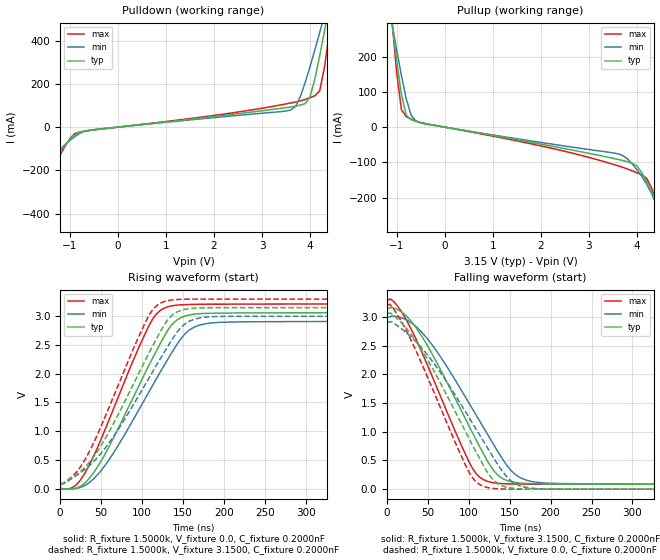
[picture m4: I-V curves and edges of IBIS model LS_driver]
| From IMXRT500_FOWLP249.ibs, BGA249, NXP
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[Model] LS_driver
|   Model LS_driver
| Library cells for typ/min/max conditions are connected as defined below:
|  pad_usbdp - External Pad
|  usb2_tx_d_data_dp - Core Input
|  gnda - gnda
|  pad_usb_vss - pad_usb_vss
|  usb2_reg_tx_fs_hiz - gnda
|  usb2_reg_tx_hs_term - gnda
|  usb2_reg_tx_hs_xcvr - gnda
|  usb2_reg_tx_ls_en - vddd
|  usbphy_d2a_txhsactive - gnda
|  vddb - vddb
|  vddd - vddd
| All other pins connected to ground
Model_type Output
Polarity   Non-Inverting
Enable   Active-Low
C_comp   2.8431pF   2.6338pF   3.0727pF
[Temperature Range]   27.0000   0.1250k   -40.0000
[Voltage Range]   3.1500V   3.0000V   3.3000V
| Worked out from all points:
|   slope of the pulldown table from 0 to 0.472 V, typ, clamps not added: 41.5 ohm
|   slope of the pullup table from 0 to 0.472 V, typ, clamps not added: 42.2 ohm
|   rising waveform, R_fixture 1.5000k, V_fixture 0.0, C_fixture 0.2000nF: 20-80 % time 64.1ns typ, 71.2ns min, 56.3ns max; typ from 0 V to 3.06 V
|   rising waveform, R_fixture 1.5000k, V_fixture 3.1500, C_fixture 0.2000nF: 20-80 % time 67.1ns typ, 75.8ns min, 57.7ns max; typ from 0.085 V to 3.15 V
|   falling waveform, R_fixture 1.5000k, V_fixture 3.1500, C_fixture 0.2000nF: 20-80 % time 66.8ns typ, 74.8ns min, 58ns max; typ from 3.15 V to 0.085 V
|   falling waveform, R_fixture 1.5000k, V_fixture 0.0, C_fixture 0.2000nF: 20-80 % time 68.9ns typ, 78.6ns min, 58.5ns max; typ from 3.06 V to 0 V
[Pulldown]
|Voltage   I(typ)   I(min)   I(max)
-3.3V     -1.789A    -1.328A    -2.415A
-2V       -541mA     -458.4mA   -672.7mA
-1.8V     -385mA     -344.5mA   -475.2mA
-1.2V     -110.9mA   -103.2mA   -128.7mA
-700mV    -18.35mA   -19.33mA   -19.54mA
3.6V      93.13mA    79.46mA    111.7mA
4V        140.3mA    280mA      135.9mA
4.2V      328.8mA    437.3mA    167.5mA
4.3V      443.1mA    519.1mA    276.2mA
4.4V      562.1mA    602.3mA    433.8mA
4.5V      683.9mA    686.7mA    605.7mA
6.6V      3.469A     2.552A     4.733A
[Pullup]
|Voltage   I(typ)   I(min)   I(max)
-3.3V     3.149A     2.232A     4.536A
-1.1V     298.4mA    297.3mA    309.5mA
-1V       188.4mA    219.5mA    155mA
-900mV    91.83mA    145.9mA    49.27mA
-800mV    33.62mA    80.51mA    29.57mA
-700mV    21.24mA    34.27mA    23.01mA
-400mV    9.525mA    9.075mA    10.13mA
3.7V      -94.61mA   -80.02mA   -113.9mA
4V        -110.4mA   -120.8mA   -129.3mA
4.2V      -153.7mA   -161.4mA   -144.6mA
4.6V      -279.6mA   -298.9mA   -297.9mA
6.6V      -2.055A    -1.587A    -2.608A
[Ramp]
| variable   typ   min   max
dV/dt_r  0.9799/85.9935n   0.8933/97.2090n   1.0678/74.5644n
dV/dt_f  0.9878/89.0736n   0.8995/0.1028u   1.0749/76.7496n
R_load = 45.0000
[Rising Waveform]
R_fixture= 1.5000k
V_fixture= 0.0
V_fixture_min= 0.0
V_fixture_max= 0.0
C_fixture= 0.2000nF
|time   V(typ)   V(min)   V(max)
0s        172.1nV    5.49uV     121.3nV
19.94ns   10.73mV    2.415mV    71.03mV
40.93ns   278.8mV    171.3mV    568mV
66.15ns   913.6mV    644.9mV    1.428V
107ns     2.113V     1.653V     2.8V
117.3ns   2.398V     1.912V     3.039V
135.3ns   2.837V     2.348V     3.179V
157.1ns   3.022V     2.758V     3.206V
193.4ns   3.055V     2.893V     3.211V
1us       3.064V     2.913V     3.215V
[Rising Waveform]
R_fixture= 1.5000k
V_fixture= 3.1500
V_fixture_min= 3.0000
V_fixture_max= 3.3000
C_fixture= 0.2000nF
|time   V(typ)   V(min)   V(max)
0s        84.94mV    86.28mV    83.78mV
22.75ns   274.8mV    254.3mV    338.8mV
47.41ns   691.8mV    573.5mV    1.002V
71.65ns   1.314V     1.05V      1.834V
108ns     2.353V     1.92V      3.009V
119.3ns   2.657V     2.193V     3.203V
131.7ns   2.946V     2.487V     3.275V
152.7ns   3.123V     2.873V     3.298V
187.5ns   3.149V     2.994V     3.3V
1us       3.15V      3V         3.3V
[Falling Waveform]
R_fixture= 1.5000k
V_fixture= 3.1500
V_fixture_min= 3.0000
V_fixture_max= 3.3000
C_fixture= 0.2000nF
|time   V(typ)   V(min)   V(max)
0s        3.15V      3V         3.3V
6.542ns   3.164V     3.018V     3.288V
18.72ns   3.079V     2.984V     3.07V
47.82ns   2.542V     2.649V     2.217V
104ns     992.2mV    1.406V     372.9mV
127.1ns   388.2mV    850.6mV    119.8mV
138.3ns   211.9mV    590.5mV    99.13mV
156.8ns   115.9mV    255.2mV    89.98mV
196.6ns   91.46mV    105mV      86.56mV
1us       84.94mV    86.28mV    83.78mV
[Falling Waveform]
R_fixture= 1.5000k
V_fixture= 0.0
V_fixture_min= 0.0
V_fixture_max= 0.0
C_fixture= 0.2000nF
|time   V(typ)   V(min)   V(max)
0s        3.064V     2.913V     3.215V
12.99ns   2.967V     2.847V     3.035V
38.09ns   2.522V     2.531V     2.327V
100.3ns   879.9mV    1.245V     294.2mV
109.6ns   628mV      1.028V     118.7mV
123.3ns   282mV      706mV      26.37mV
133.9ns   112.6mV    464.2mV    7.693mV
151ns     20.17mV    152.3mV    922.5uV
185.7ns   411.8uV    6.602mV    33.55uV
1us       195.5nV    5.899uV    129.1nV
